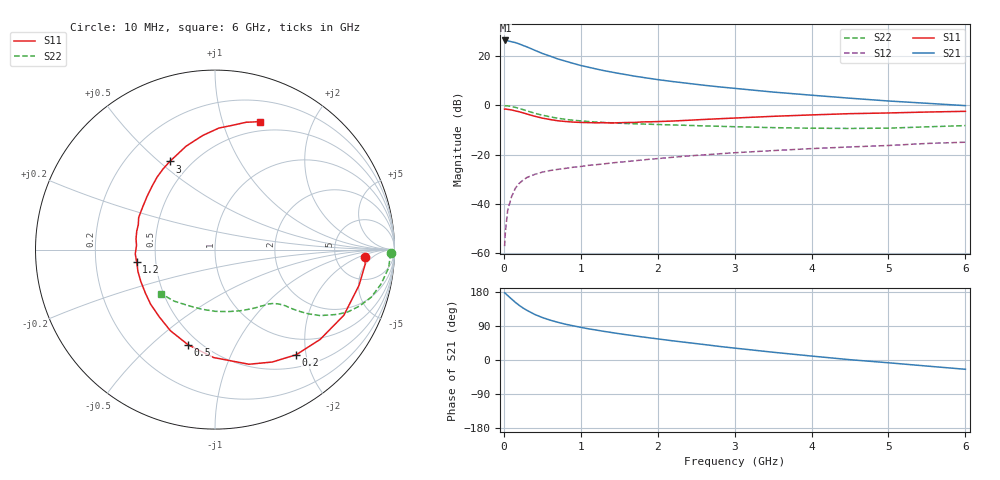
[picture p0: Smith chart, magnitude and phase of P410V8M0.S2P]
! SIEMENS Small Signal Semiconductors
! BFP182
! Si NPN RF Bipolar Junction Transistor in SOT143
! VCE = 10 V  IC = 8 mA
! Common Emitter S-Parameters:  March  1996
# GHz  S  MA  R  50
!  f  S11  S21  S12  S22
! GHz  MAG  ANG  MAG  ANG  MAG  ANG  MAG  ANG
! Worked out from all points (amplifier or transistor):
!   36 points, 10 MHz to 6 GHz, reference 50 ohm
!   highest |S21| = 26.3 dB at 20 MHz (marker M1)
!   |S21| within 3 dB of that: start of sweep to 329.5 MHz
!   unconditionally stable (mu >= 1): 1.421 GHz to 5.725 GHz
!   at 250 MHz: K = 0.28, MSG = 27.3 dB, |S12| = -30.3 dB
!   at 1.4 GHz: K = 0.99, MSG = 18.4 dB, |S12| = -23.4 dB
!   at 6 GHz: K = 0.97, MSG = 7.4 dB, |S12| = -15.0 dB
!   S11 on the Smith chart (normalised r, x): 10 MHz: 10, -3; 200 MHz: 0.70, -1.82; 500 MHz: 0.43, -0.66; 1.2 GHz: 0.39, -0.07; 3 GHz: 0.38, +0.54; 6 GHz: 0.40, +1.33
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0.01  0.8354 -2.8  20.38 177.3  0.0014 78.8  0.9818 -1.1
0.02  0.8406 -5.6  20.61 176.0  0.0027 76.8  0.976 -2.4
0.05  0.8269 -13.9  20.26 170.1  0.0075 85.4  0.973 -6.0
0.1  0.8058 -27.0  19.41 161.0  0.014 74.7  0.9444 -11.8
0.15  0.7705 -40.5  18.66 152.1  0.0209 68.4  0.9096 -17.0
0.2  0.7402 -52.3  17.54 144.2  0.0262 64.5  0.8647 -21.3
0.25  0.703 -63.0  16.31 137.1  0.0305 59.0  0.8193 -25.0
0.3  0.6662 -73.5  15.27 131.1  0.0345 55.5  0.7717 -27.9
0.4  0.6013 -90.8  13.09 120.4  0.0398 50.3  0.6919 -32.1
0.5  0.551 -105.8  11.25 112.1  0.0443 46.1  0.6321 -34.5
0.6  0.5158 -118.8  9.944 105.3  0.0477 44.2  0.5848 -36.1
0.7  0.4864 -129.8  8.715 99.6  0.0503 42.6  0.5479 -37.3
0.9  0.4572 -148.1  7.078 90.3  0.0556 41.3  0.4983 -38.7
1.1  0.4462 -164.1  5.918 82.3  0.0607 40.8  0.4696 -40.3
1.2  0.4418 -171.0  5.448 79.1  0.0627 40.4  0.4583 -41.2
1.7  0.4492 162.1  3.896 63.8  0.0754 40.5  0.4213 -46.2
2.2  0.4806 142.0  3.023 50.5  0.0887 38.7  0.3999 -53.2
3  0.552 117.1  2.206 31.4  0.1094 34.3  0.3686 -67.6
3.5  0.5984 105.6  1.856 20.5  0.121 30.9  0.353 -78.2
4.5  0.6774 88.2  1.393 0.8  0.1434 24.1  0.3402 -102.8
5.5  0.7306 76.2  1.099 -16.0  0.1688 17.8  0.3663 -128.3
6  0.7557 70.6  0.985 -24.5  0.1788 13.5  0.3883 -140.7
